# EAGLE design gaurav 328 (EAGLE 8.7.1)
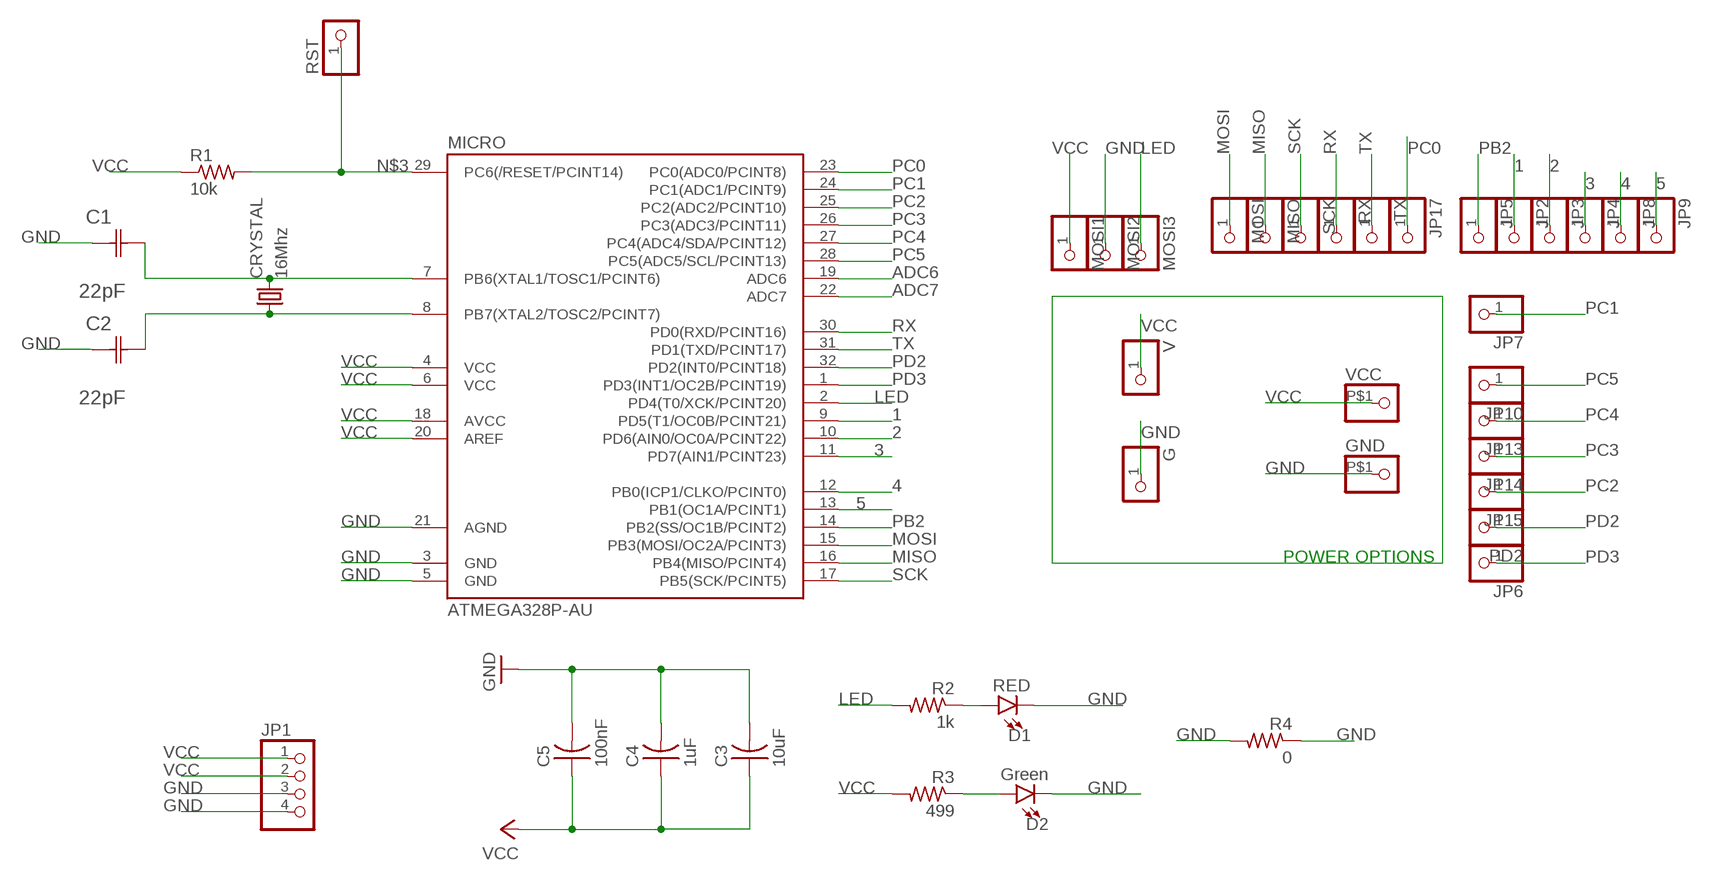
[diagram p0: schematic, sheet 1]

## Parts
C1  22pF  0612ZC225MAT2A  [CAPC3216X178N]
C2  22pF  0612ZC225MAT2A  [CAPC3216X178N]
C3  10uF  CAP-US1206FAB  [C1206FAB]
C4  1uF  CAP-US1206FAB  [C1206FAB]
C5  100nF  CAP-US1206FAB  [C1206FAB]
CRYSTAL  16Mhz  CSM-7X-DU  [CSM-7X-DU]
D1  RED  LED-RED1206  [LED-1206]
D2  Green  LED-RED1206  [LED-1206]
G  PINHD-1X1  [1X01]
GND  PINHD-1X1-BIGPOGO  [1X1-BIGPOGO]
JP1  PINHD-1X4  [1X04]
JP2  PINHD-1X1  [1X01]
JP3  PINHD-1X1  [1X01]
JP4  PINHD-1X1  [1X01]
JP5  PINHD-1X1  [1X01]
JP6  PINHD-1X1  [1X01]
JP7  PINHD-1X1  [1X01]
JP8  PINHD-1X1  [1X01]
JP9  PINHD-1X1  [1X01]
JP10  PINHD-1X1  [1X01]
JP13  PINHD-1X1  [1X01]
JP14  PINHD-1X1  [1X01]
JP15  PINHD-1X1  [1X01]
JP17  PINHD-1X1  [1X01]
MICRO  ATMEGA328P-AU  ATMEGA48/88/168-AU  [TQFP32-08]
MISO  PINHD-1X1  [1X01]
MOSI  PINHD-1X1  [1X01]
MOSI1  PINHD-1X1  [1X01]
MOSI2  PINHD-1X1  [1X01]
MOSI3  PINHD-1X1  [1X01]
PD2  PINHD-1X1  [1X01]
R1  10k  RES-US1206FAB  [R1206FAB]
R2  1k  RES-US1206FAB  [R1206FAB]
R3  499  RES-US1206FAB  [R1206FAB]
R4  0  RES-US1206FAB  [R1206FAB]
RST  PINHD-1X1  [1X01]
RX  PINHD-1X1  [1X01]
SCK  PINHD-1X1  [1X01]
TX  PINHD-1X1  [1X01]
V  PINHD-1X1  [1X01]
VCC  PINHD-1X1-BIGPOGO  [1X1-BIGPOGO]

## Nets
1: JP2.1 MICRO.9(PD5(T1/OC0B/PCINT21))
2: JP3.1 MICRO.10(PD6(AIN0/OC0A/PCINT22))
3: JP4.1 MICRO.11(PD7(AIN1/PCINT23))
4: JP8.1 MICRO.12(PB0(ICP1/CLKO/PCINT0))
5: JP9.1 MICRO.13(PB1(OC1A/PCINT1))
ADC6: MICRO.19(ADC6)
ADC7: MICRO.22(ADC7)
GND: C1.1(C1) C2.1(C1) C3.2 C4.2 C5.2 D1.C D2.C G.1 GND.P$1 JP1.3 JP1.4 MICRO.3(GND) MICRO.5(GND) MICRO.21(AGND) MOSI2.1 R4.1 R4.2
LED: MICRO.2(PD4(T0/XCK/PCINT20)) MOSI3.1 R2.2
MISO: MICRO.16(PB4(MISO/PCINT4)) MISO.1
MOSI: MICRO.15(PB3(MOSI/OC2A/PCINT3)) MOSI.1
N$1: D2.A R3.1
N$2: C1.2(C2) CRYSTAL.2 MICRO.7(PB6(XTAL1/TOSC1/PCINT6))
N$3: MICRO.29(PC6(/RESET/PCINT14)) R1.2 RST.1
N$9: C2.2(C2) CRYSTAL.1 MICRO.8(PB7(XTAL2/TOSC2/PCINT7))
N$25: D1.A R2.1
PB2: JP5.1 MICRO.14(PB2(SS/OC1B/PCINT2))
PC0: JP17.1 MICRO.23(PC0(ADC0/PCINT8))
PC1: JP7.1 MICRO.24(PC1(ADC1/PCINT9))
PC2: JP15.1 MICRO.25(PC2(ADC2/PCINT10))
PC3: JP14.1 MICRO.26(PC3(ADC3/PCINT11))
PC4: JP13.1 MICRO.27(PC4(ADC4/SDA/PCINT12))
PC5: JP10.1 MICRO.28(PC5(ADC5/SCL/PCINT13))
PD2: MICRO.32(PD2(INT0/PCINT18)) PD2.1
PD3: JP6.1 MICRO.1(PD3(INT1/OC2B/PCINT19))
RX: MICRO.30(PD0(RXD/PCINT16)) RX.1
SCK: MICRO.17(PB5(SCK/PCINT5)) SCK.1
TX: MICRO.31(PD1(TXD/PCINT17)) TX.1
VCC: C3.1 C4.1 C5.1 JP1.1 JP1.2 MICRO.4(VCC) MICRO.6(VCC) MICRO.18(AVCC) MICRO.20(AREF) MOSI1.1 R1.1 R3.2 V.1 VCC.P$1

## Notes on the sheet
- POWER OPTIONS

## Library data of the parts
C1 C2 = AVX_By_element14_Batch_1:0612ZC225MAT2A: Capacitor 1206; MPN: 0612ZC225MAT2A; OC_FARNELL: -; OC_NEWARK: 12N3209; SUPPLIER: AVX; TOLERANCE: ±20%; VALUE: 2.2µF; VOLTAGERATING: 10V
C3-C5 = fab:CAP-US
CRYSTAL = 01_FAB_Hello:CSM-7X-DU: SMD CRYSTAL; OC_FARNELL: unknown; OC_NEWARK: unknown
D1 = SparkFun-LED:LED-RED: Red SMD LED; PROD_ID: DIO-09912
D2 = SparkFun-LED:LED-RED: Red SMD LED; PROD_ID: DIO-09912; VALUE: RED
G GND JP2-JP10 JP13-JP15 JP17 MISO MOSI MOSI1-MOSI3 PD2 RST RX SCK TX V VCC = adafruit:PINHD-1X1: Pin header 1x1 for 0.1" spacing
JP1 = pinhead:PINHD-1X4: PIN HEADER
MICRO = atmega8:ATMEGA48/88/168
R1-R4 = fab:RES-US: Resistor (US Symbol)

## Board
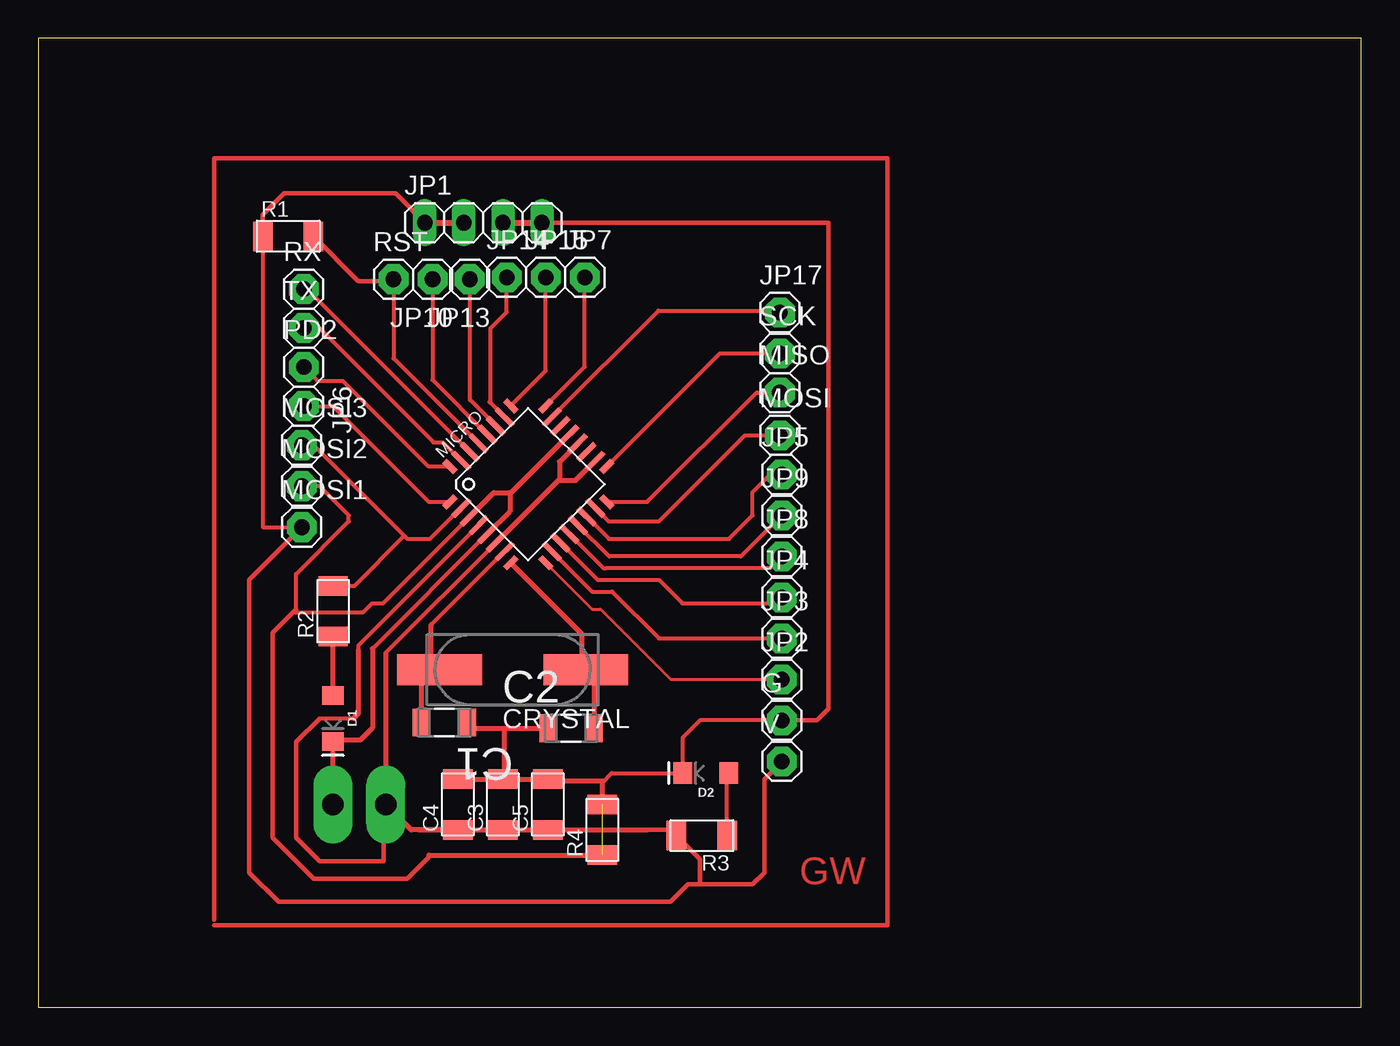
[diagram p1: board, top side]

Size 86.09 x 63.04 mm. Coordinates in mm from the lower left corner, seen from the top.
Outline: 0,0 86.09,0 86.09,63.04 0,63.04 0,0
Copper layers (1*16): Top 0.035mm / dielectric 1.5mm / Bottom 0.035mm
Design rules "fab (1)": minimum track width 0.3mm, minimum drill 32mil, track to track 0.315mm, track to pad 0.315mm, pad to pad 0.315mm, via to via 0.315mm, smd to smd 0.315mm, copper to edge 40mil, drill to drill 16mil, minimum pad ring 10mil, minimum via ring 8mil, stop-mask expansion 4mil, vias tented up to drill 0mil, thermal gap 10mil

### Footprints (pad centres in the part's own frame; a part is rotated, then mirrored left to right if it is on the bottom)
CAPC3216X178N = smd 1.118 x 1.803: 1 -1.499,0; 2 1.499,0
C1206FAB = smd 1.27 x 1.905: 1 -1.651,0; 2 1.651,0
CSM-7X-DU = smd 5.5 x 2: 1 -4.75,0; 2 4.75,0
LED-1206 = smd 1.2 x 1.4: A -1.5,0; C 1.5,0
1X01 = drill 1.016 pad 1.93 octagon: 1 0,0
1X1-BIGPOGO = drill 1.4 pad 2.54 long: P$1 0,0
1X04 = drill 1.016 long: 1 -3.81,0; 2 -1.27,0; 3 1.27,0; 4 3.81,0
TQFP32-08 = smd 1.016 x 0.406: 1 -4.42,2.8; 8 -4.42,-2.8; 17 4.42,-2.8; 24 4.42,2.8 | smd 1.524 x 0.356: 2 -4.166,2; 3 -4.166,1.2; 4 -4.166,0.4; 5 -4.166,-0.4; 6 -4.166,-1.2; 7 -4.166,-2; 18 4.166,-2; 19 4.166,-1.2; 20 4.166,-0.4; 21 4.166,0.4; 22 4.166,1.2; 23 4.166,2 | smd 0.406 x 1.016: 9 -2.8,-4.42; 16 2.8,-4.42; 25 2.8,4.42; 32 -2.8,4.42 | smd 0.356 x 1.524: 10 -2,-4.166; 11 -1.2,-4.166; 12 -0.4,-4.166; 13 0.4,-4.166; 14 1.2,-4.166; 15 2,-4.166; 26 2,4.166; 27 1.2,4.166; 28 0.4,4.166; 29 -0.4,4.166; 30 -1.2,4.166; 31 -2,4.166
R1206FAB = smd 1.27 x 1.905: 1 -1.651,0; 2 1.651,0

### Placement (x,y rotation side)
C1  26.42,18.54 180 top
C2  34.67,18.16 0 top
C3  30.23,13.21 90 top
C4  27.3,13.21 90 top
C5  33.15,13.21 90 top
CRYSTAL  30.86,21.97 180 top
D1  19.18,18.8 270 top
D2  43.43,15.24 180 top
G  48.39,18.67 0 top
GND  19.18,13.21 90 top
JP1  28.96,51.05 0 top
JP2  48.39,21.34 0 top
JP3  48.39,24 0 top
JP4  48.39,26.67 0 top
JP5  48.39,34.67 0 top
JP6  17.27,39.12 269.6 top
JP7  35.56,47.5 0 top
JP8  48.39,29.34 0 top
JP9  48.39,32 0 top
JP10  25.65,47.37 180 top
JP13  28.07,47.37 180 top
JP14  30.48,47.5 0 top
JP15  33.02,47.5 0 top
JP17  48.26,45.21 0 top
MICRO  31.88,34.04 45 top
MISO  48.26,40 0 top
MOSI  48.26,37.21 0 top
MOSI1  17.15,31.24 0 top
MOSI2  17.15,33.91 0 top
MOSI3  17.15,36.58 0 top
PD2  17.27,41.66 0 top
R1  16.26,50.17 0 top
R2  19.18,25.78 90 top
R3  43.18,11.18 180 top
R4  36.7,11.56 90 top
RST  23.11,47.37 0 top
RX  17.27,46.74 0 top
SCK  48.26,42.55 0 top
TX  17.27,44.2 0 top
V  48.39,16 0 top
VCC  22.61,13.21 90 top

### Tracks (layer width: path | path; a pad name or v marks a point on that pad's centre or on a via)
1
  Top 0.203: MICRO.9 36.05,25.91 36.58,25.91 41.15,21.34 JP2.1
2
  Top 0.254: MICRO.10 36.03,27.05 37.34,27.05 40.39,24 JP3.1 49.15,24
3
  Top 0.254: JP4.1 48.2,26.48 48.01,26.29 41.91,26.29 40.39,27.81 36.4,27.81 MICRO.11
4
  Top 0.254: 48.01,28.57 48.01,28.96 JP8.1 47.62,28.57 36.96,28.57 36.77,28.57 MICRO.12
5
  Top 0.254: JP9.1 45.72,29.34 37.14,29.34 MICRO.13
GND  (1 unrouted)
  Top 0.254: G.1 48.01,18.67 43.05,18.67 41.93,17.55 D2.C 37.31,15.24 36.7,14.63 | 16.76,25.91 16.76,28.19 20.19,31.62 20.19,32 18.29,33.91 MOSI2.1 | 16.57,25.72 21.15,25.72 21.72,26.29 22.43,26.29 28.36,32.22 | MICRO.5 21.75,23.34
  Top 0.305: 48.01,18.67 50.67,18.67 51.44,19.43 51.44,51.05 JP1.4 | 16.76,25.91 16.57,25.72 15.24,24.38 15.24,11.05 17.91,8.38 24,8.38 25.4,9.78 25.4,9.91
  Top 0.33: 18.95,17.3 D1.C | D1.C 18.8,16.91 | MICRO.3 28.36,32.22 29.63,33.49 30.69,33.49 | C1.1 28.3,18.16 30.35,18.16 | 30.35,18.16 C2.1 | GND.P$1 D1.C | D1.C 19.28,17.4 20.95,17.4 21.75,18.19 21.75,23.34 | 25.4,9.91 R4.1 | C3.2 30.1,14.99 | C4.2 C3.2 | C3.2 C5.2 32.77,14.73 36.8,14.73 36.7,14.63 R4.2 | C3.2 30.35,14.99 30.35,18.16 | 30.69,33.49 30.69,32.29 MICRO.5 | MICRO.21 30.76,33.49 30.69,33.49
  Top 0.406: JP1.3 JP1.4
LED
  Top 0.254: MOSI3.1 17.91,36.58 23.81,30.67 | 23.81,30.67 24,30.48 25.49,30.48 MICRO.2 | R2.2 20.57,27.43 23.81,30.67
MISO
  Top 0.254: MISO.1 46.74,40 39.62,32.89 MICRO.16
MOSI
  Top 0.254: MOSI.1 45.97,37.21 40.39,31.62 37.12,31.62 MICRO.15
N$1
  Top 0.254: R3.1 44.83,15.14 D2.A
N$2
  Top 0.254: 25.57,24.9 MICRO.7
  Top 0.33: CRYSTAL.2 25.57,21.54 | 25.57,21.54 24.89,21.01 24.89,18.03 24.92,18.06 C1.2 | 25.57,21.54 25.57,24.9
N$3
  Top 0.254: MICRO.29 23.11,42.23 RST.1
  Top 0.305: RST.1 23.11,47.24 20.93,47.24 arc-45 20.75,47.32 R1.2
N$6
  Top 0.305: 11.43,5.33 55.25,5.33 55.25,55.25 11.43,55.25 11.43,5.71
N$9
  Top 0.33: MICRO.8 35.36,24.31 35.36,22.22 CRYSTAL.1 36.17,21.16 C2.2
N$25
  Top 0.33: D1.A R2.1
PB2
  Top 0.254: JP5.1 47.62,34.67 46.48,33.53 46.48,32 44.96,30.48 37.34,30.48 37.13,30.48 MICRO.14
PC0
  Top 0.254: 33.44,38.4 MICRO.23 40.35,45.34 48.13,45.34 JP17.1
PC1
  Top 0.254: JP7.1 35.56,41.68 MICRO.24
PC2
  Top 0.254: JP15.1 33.02,41.43 MICRO.25
PC3
  Top 0.254: MICRO.26 29.42,39.32 | 29.42,39.32 29.34,39.4 | 29.42,39.32 29.42,44.17 30.48,45.23 JP14.1
PC4
  Top 0.254: MICRO.27 28.09,39.52 | 28.09,39.52 28.07,39.54 | 28.09,39.52 28.09,47.35 JP13.1
PC5
  Top 0.254: MICRO.28 25.65,40.83 JP10.1
PD2
  Top 0.254: PD2.1 18.16,40.77 19.81,40.77 25.4,35.18 MICRO.32
PD3
  Top 0.254: JP6.1 19.18,39.12 25.4,32.89 MICRO.1
RX
  Top 0.254: MICRO.30 17.53,46.69 17.53,46.74
  Top 0.305: RX.1 17.53,46.74 17.65,46.74
SCK
  Top 0.254: MICRO.17 44.35,42.55 SCK.1
TX
  Top 0.254: TX.1 18.29,44.2 25.72,36.77 26.32,36.77 MICRO.31
VCC
  Top 0.254: R1.1 14.6,31.24 MOSI1.1 | 20.49,18.8 18.29,18.8 | MICRO.6 22.61,23.07 | 20.83,23.24 20.83,23.55 MICRO.4
  Top 0.305: R1.1 14.6,51.56 16,52.96 23.24,52.96 JP1.1 | 18.29,18.8 16.76,17.27 16.76,11.05 18.29,9.52 22.48,9.52 22.48,13.59 22.61,13.72 | MOSI1.1 13.72,27.81 13.72,8.76 15.62,6.86 41.15,6.86 42.29,8 43.05,8 | 39.62,11.56 41.15,11.56 R3.2 43.05,9.65 43.05,8 | 43.05,8 46.48,8 47.24,8.76 47.24,14.86 V.1
  Top 0.33: C4.1 C3.1 C5.1 39.62,11.56 | 24.77,11.56 C4.1 | 20.49,18.8 20.83,19.14 20.83,23.24 | C4.1 24.26,11.56 VCC.P$1 | MICRO.20 33.91,35.5 33.91,34.37 | 33.91,34.37 33.91,34.29 34.96,34.29 MICRO.18 | MICRO.6 33.91,34.37 | 22.61,23.07 22.61,13.72 VCC.P$1 | VCC.P$1 22.48,13.08
  Top 0.406: JP1.1 JP1.2

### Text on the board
Top: GW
